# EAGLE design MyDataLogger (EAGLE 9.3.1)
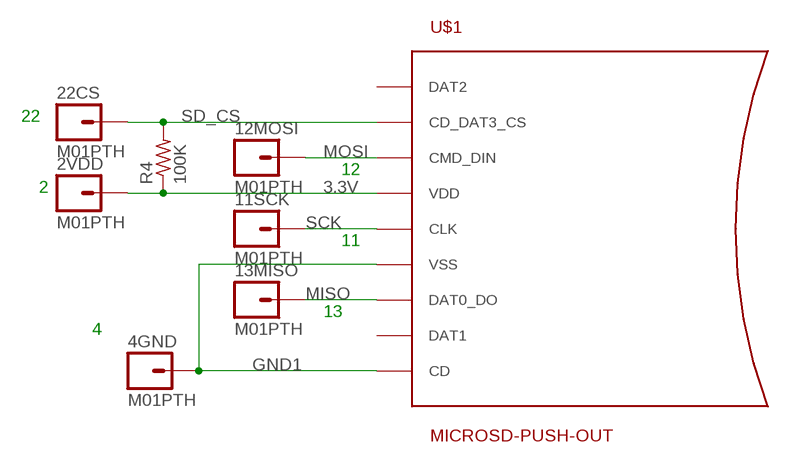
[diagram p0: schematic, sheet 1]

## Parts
2VDD  M01PTH  [1X01]
4GND  M01PTH  [1X01]
11SCK  M01PTH  [1X01]
12MOSI  M01PTH  [1X01]
13MISO  M01PTH  [1X01]
22CS  M01PTH  [1X01]
R4  100K  R-US_0204/7  [0204/7]
U$1  MICROSD-PUSH-OUT  [MICROSD-PUSH-OUT]

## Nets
3.3V: 2VDD.1 R4.1 U$1.4(VDD)
GND1: 4GND.1 U$1.6(VSS) U$1.CD U$1.G1(VSS) U$1.G2(VSS) U$1.G3(VSS) U$1.G4(VSS)
MISO: 13MISO.1 U$1.7(DAT0_DO)
MOSI: 12MOSI.1 U$1.3(CMD_DIN)
SCK: 11SCK.1 U$1.5(CLK)
SD_CS: 22CS.1 R4.2 U$1.2(CD_DAT3_CS)
Unconnected: U$1.1(DAT2) U$1.8(DAT1)

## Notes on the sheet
- 22
- 12
- 2
- 11
- 13
- 4

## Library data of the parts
2VDD 4GND 11SCK 12MOSI 13MISO 22CS = SparkFun-Connectors:M01: Header 1
R4 = rcl:R-US_: RESISTOR, American symbol; SPICEPREFIX: R
U$1 = microsd:MICROSD-PUSH-OUT: T-Flash Push-Out Micro SD Card Reader 14.75mm x 14.5mm SMD with external pins

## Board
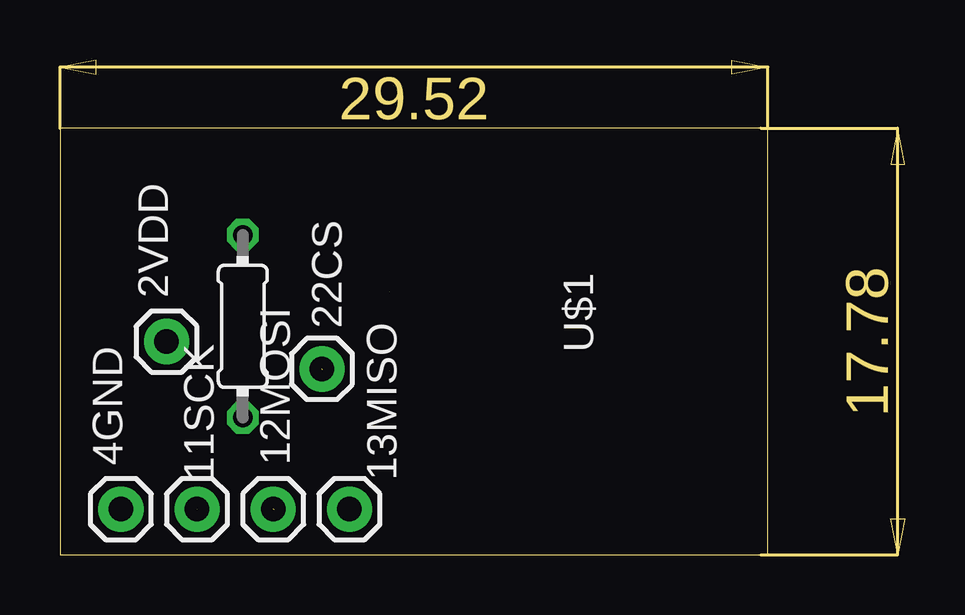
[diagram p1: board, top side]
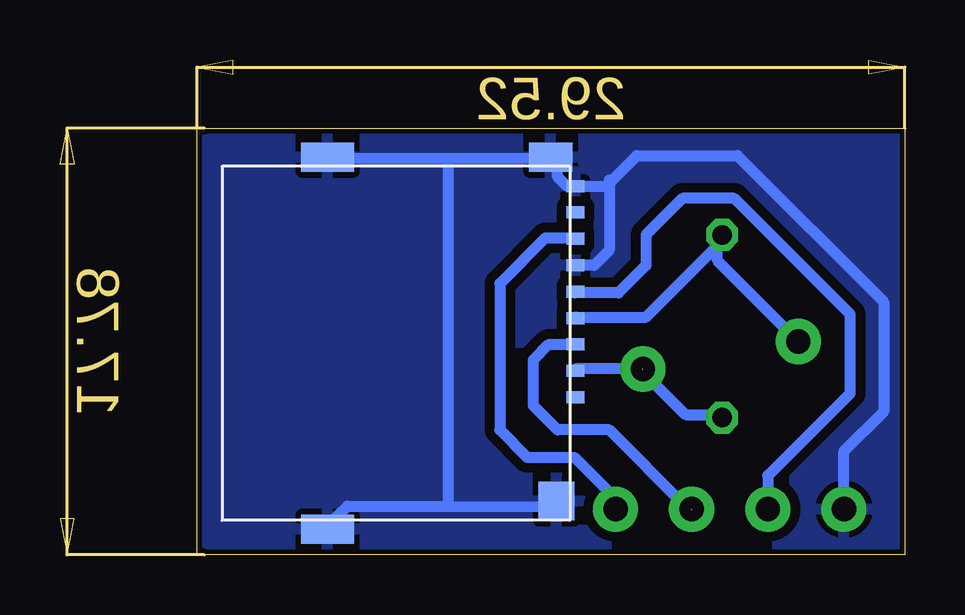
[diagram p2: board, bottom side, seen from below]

Size 35.22 x 20.62 mm. Coordinates in mm from the lower left corner, seen from the top.
Outline: 0,0 29.52,0 29.52,17.77 0,17.77 0,0
Copper layers (1*16): Top 0.035mm / dielectric 1.5mm / Bottom 0.035mm
Design rules "MTS *": minimum track width 18mil, minimum drill 12mil, track to track 16mil, track to pad 12mil, pad to pad 6mil, via to via 6mil, smd to smd 0mil, copper to edge 8mil, drill to drill 10mil, minimum pad ring 10mil, minimum via ring 10mil, stop-mask expansion 2mil, vias tented up to drill 25mil, thermal gap 10mil

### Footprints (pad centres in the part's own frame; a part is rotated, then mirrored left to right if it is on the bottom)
1X01 = drill 1.016 pad 1.88: 1 0,0
0204/7 = drill 0.813 octagon: 1 -3.81,0; 2 3.81,0
MICROSD-PUSH-OUT = smd 0.5 x 0.75: 1 9.625,0.225; 2 8.525,0.225; 3 7.425,0.225; 4 6.325,0.225; 5 5.225,0.225; 6 4.125,0.225; 7 3.025,0.225; 8 1.925,0.225; CD 0.825,0.225 | smd 1.2 x 1.8: G1 -0.375,-0.8 | smd 1.2 x 2.2: G2 -0.375,-10.1; G4 15.125,-10.1 | smd 1.6 x 1.5: G3 13.95,-0.55

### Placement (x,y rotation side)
2VDD  4.45,8.89 0 top
4GND  2.54,1.91 0 top
11SCK  5.71,1.91 0 top
12MOSI  8.89,1.91 0 top
13MISO  12.06,1.91 0 top
22CS  10.92,7.75 0 top
R4  7.62,9.53 270 top
U$1  13.97,16.19 270 bottom

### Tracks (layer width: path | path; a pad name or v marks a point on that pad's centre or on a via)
3.3V
  Bottom 0.457: U$1.4 13.71,9.91 10.79,9.91 7.81,12.89 | 7.81,12.89 7.62,13.08 R4.1 | 7.81,12.89 7.81,12.26 2VDD.1
GND1
  Bottom 0.457: 4GND.1 2.54,4.32 0.89,5.97 0.89,10.54 6.99,16.64 11.18,16.64 12.32,15.49 12.32,15.37 13.72,15.37 U$1.CD 14.1,15.37 14.48,15.75 14.48,16.54 14.77,16.54 | 19.05,2.03 23.24,2.03 24.04,1.27 24.04,1.07 | 19.05,2.03 14.83,2 14.55,2.27 | 12.32,15.62 12.32,12.7 12.95,12.06 U$1.6 | 19.05,16.51 14.86,16.51 U$1.G1 | 19.05,16.51 24,16.51 U$1.G2 | 19.05,16.51 19.05,2.03
  pour Bottom: 0,0 29.21,0 29.21,17.78 0,17.78
MISO
  Bottom 0.457: U$1.7 13.79,13.21 14.99,13.21 16.89,11.3 16.89,5.21 15.75,4.06 13.78,4.06 12.06,2.35 13MISO.1
MOSI  (1 unrouted)
  Bottom 0.457: 8.92,1.87 9.14,2.03 12.32,5.21 14.48,5.21 15.49,6.22 15.49,8.13 14.85,8.77 U$1.3
SCK  (2 unrouted)
  Bottom 0.457: U$1.5 13.74,10.92 11.94,10.92 10.79,12.06 10.79,13.34 9.27,14.86 7.11,14.86 2.29,10.03 2.29,6.73 5.71,3.3 11SCK.1
SD_CS  (3 unrouted)
  Bottom 0.457: 22CS.1 13.73,7.75 13.73,7.67 | R4.2 7.62,5.84 9.14,5.84 10.79,7.49 10.95,7.71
